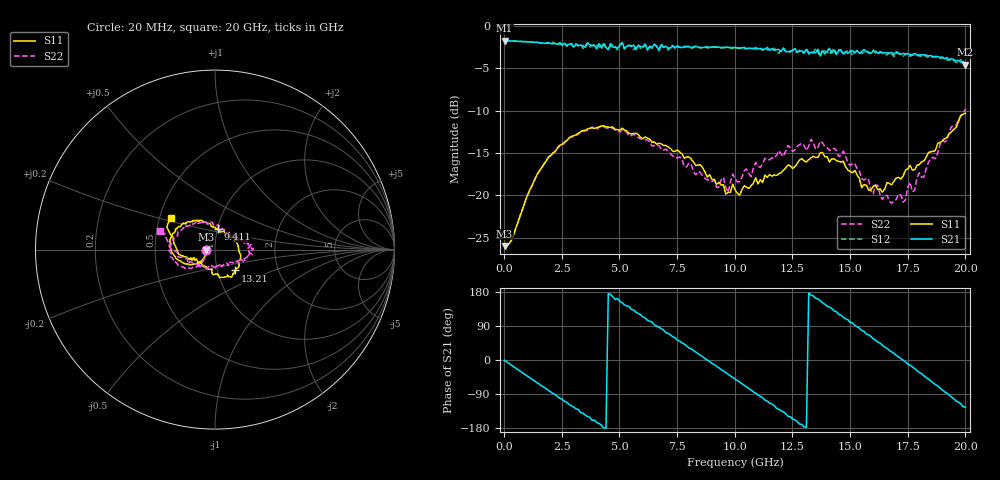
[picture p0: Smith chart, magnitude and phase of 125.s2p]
!Agilent Technologies,N5230A,US43500223,A.07.50.48
!Agilent N5230A: A.07.50.48
!Date: Tuesday, September 15, 2015 20:14:11
!Correction: S11(Full 2 Port(1,2))
!S21(Full 2 Port(1,2))
!S12(Full 2 Port(1,2))
!S22(Full 2 Port(1,2))
!S2P File: Measurements: S11, S21, S12, S22:
# Hz S  dB  R 50
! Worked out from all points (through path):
!   201 points, 20 MHz to 20 GHz, reference 50 ohm
!   highest |S21| = -1.72 dB at 20 MHz (marker M1); lowest = -4.6 dB at 20 GHz (marker M2)
!   group delay of S21, straight-line fit = 116 ps
!   lowest |S11| = -26.0 dB at 20 MHz (marker M3), VSWR 1.11, Z = 45.2 - j0.0134 ohm
!   |S11| at or under -10 dB: start of sweep to end of sweep
!   |S22| runs from -26.0 to -9.8 dB; largest |S21 - S12| = 0.059
!   S11 on the Smith chart (normalised r, x): 20 MHz: 0.90, -0.00; 9.411 GHz: 1.01, +0.23; 13.21 GHz: 1.22, -0.29; 20 GHz: 0.57, +0.23
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2e7  -25.98 -179.8  -1.72 -0.9  -1.72 -1.0  -26.01 -179.4
9.191e8  -20.67 -140.9  -1.84 -38.9  -1.86 -38.9  -20.65 -136.0
1.9181e9  -15.49 -150.1  -1.95 -80.2  -1.97 -80.8  -15.54 -141.2
3.4166e9  -12.37 -177.2  -2.31 -140.1  -2.66 -139.7  -12.38 -163.3
4.3157e9  -11.80 165.7  -2.25 -179.3  -1.91 -177.3  -11.90 179.7
5.1149e9  -12.07 152.6  -1.95 151.3  -2.04 150.4  -12.25 163.8
6.1139e9  -13.11 137.6  -2.13 111.1  -2.17 112.8  -13.45 144.7
6.7133e9  -13.85 126.3  -2.92 86.7  -2.86 86.3  -14.15 132.1
8.012e9  -15.47 112.5  -2.48 31.8  -2.40 31.9  -16.22 98.5
9.4106e9  -18.81 81.3  -2.55 -25.2  -2.58 -25.8  -18.16 50.6
1.001e10  -19.33 60.3  -2.54 -50.0  -2.55 -50.8  -17.99 38.1
1.09091e10  -17.94 31.3  -2.56 -87.5  -2.76 -88.1  -16.12 23.7
1.17083e10  -17.60 3.2  -2.89 -120.1  -2.62 -120.9  -15.63 12.3
1.26074e10  -16.62 -27.9  -2.67 -158.2  -3.11 -159.2  -14.66 9.9
1.32068e10  -15.80 -45.7  -3.31 176.4  -3.17 173.0  -14.22 3.2
1.34066e10  -15.38 -52.2  -3.12 168.9  -3.20 171.5  -13.79 -1.1
1.5005e10  -17.17 -83.1  -2.98 99.1  -2.88 98.3  -16.49 -23.3
1.56044e10  -18.75 -106.5  -2.79 75.5  -3.14 75.2  -18.21 -36.0
1.67033e10  -18.59 -148.2  -3.25 25.2  -3.12 25.4  -20.68 -64.3
1.78022e10  -16.97 -160.5  -3.25 -22.7  -3.40 -23.0  -19.41 -125.1
1.86014e10  -14.82 -169.3  -3.63 -60.3  -3.66 -60.9  -15.53 -153.1
2e10  -10.31 144.1  -4.56 -124.9  -4.69 -126.7  -9.84 161.5
